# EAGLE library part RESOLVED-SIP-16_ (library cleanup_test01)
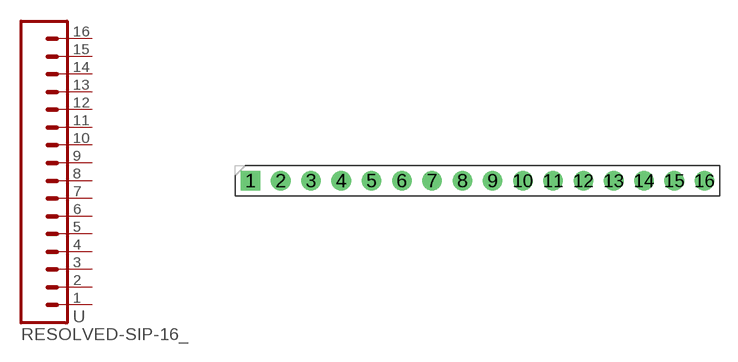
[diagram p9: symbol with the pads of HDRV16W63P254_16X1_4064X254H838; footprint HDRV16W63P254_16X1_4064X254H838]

Designator prefix -

## RESOLVED-SIP-16_2.54-SPACE-VERTICAL  [HDRV16W63P254_16X1_4064X254H838]
1  1  pas
2  2  pas
3  3  pas
4  4  pas
5  5  pas
6  6  pas
7  7  pas
8  8  pas
9  9  pas
10  10  pas
11  11  pas
12  12  pas
13  13  pas
14  14  pas
15  15  pas
16  16  pas

## Footprint HDRV16W63P254_16X1_4064X254H838 (pad centres in mm)
drill 1.1 pad 1.65 square: 1 0,0
drill 1.1 pad 1.65: 2 2.54,0; 3 5.08,0; 4 7.62,0; 5 10.16,0; 6 12.7,0; 7 15.24,0; 8 17.78,0; 9 20.32,0; 10 22.86,0; 11 25.4,0; 12 27.94,0; 13 30.48,0; 14 33.02,0; 15 35.56,0; 16 38.1,0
